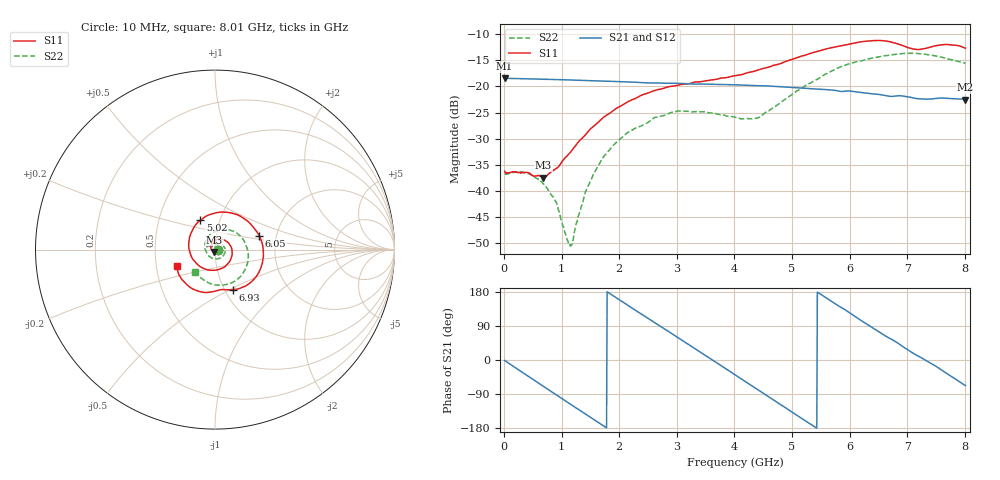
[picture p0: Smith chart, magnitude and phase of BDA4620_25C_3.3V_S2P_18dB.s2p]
!Agilent Technologies,E5071B,MY42404982,A.09.10
!Date: Wed May 06 08:52:32 2026
!Data & Calibration Information:
!Freq	S11:SOLT2(ON)	S21:SOLT2(ON)	S12:SOLT2(ON)	S22:SOLT2(ON)
# Hz S RI R 50
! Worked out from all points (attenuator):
!   801 points, 10 MHz to 8.01 GHz, reference 50 ohm
!   highest |S21| = -18.41 dB at 10 MHz (marker M1); lowest = -22.5 dB at 8.01 GHz (marker M2)
!   lowest |S11| = -37.5 dB at 680 MHz (marker M3), VSWR 1.03, Z = 49.7 - j1.3 ohm
!   |S11| at or under -10 dB: start of sweep to end of sweep
!   |S22| runs from -50.6 to -13.6 dB; largest |S21 - S12| = 0.00059
!   S11 on the Smith chart (normalised r, x): 10 MHz: 1.03, -0.00; 5.02 GHz: 0.81, +0.27; 6.05 GHz: 1.62, +0.27; 6.93 GHz: 1.09, -0.52; 8.01 GHz: 0.64, -0.13
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1e7  0.0154 -0.00104  0.1201 -0.00251  0.1202 -0.00259  0.0144 -0.00056
4.2e8  0.00861 -0.0122  0.0866 -0.0804  0.0867 -0.0806  0.0136 -0.00548
6.8e8  -0.00279 -0.0131  0.0418 -0.1096  0.0419 -0.1097  0.00894 -0.00752
8.9e8  -0.0137 -0.0086  -0.000386 -0.1163  -0.000431 -0.1166  0.00341 -0.00727
1.14e9  -0.0222 0.0058  -0.0492 -0.1043  -0.0494 -0.1044  -0.00257 -0.00184
1.19e9  -0.023 0.0098  -0.058 -0.0993  -0.0582 -0.0995  -0.00329 -8.74e-05
1.35e9  -0.0227 0.0223  -0.0827 -0.0789  -0.0827 -0.079  -0.00497 0.0053
1.58e9  -0.0135 0.0404  -0.1058 -0.0402  -0.1059 -0.0403  -0.0041 0.0148
1.87e9  0.0119 0.0559  -0.1107 0.0155  -0.1109 0.0156  0.00411 0.0259
2.16e9  0.0458 0.0553  -0.0885 0.0662  -0.0885 0.0661  0.0189 0.0312
2.68e9  0.0935 0.00364  -0.00434 0.1077  -0.0043 0.1079  0.0474 0.0193
3.08e9  0.0838 -0.0625  0.0642 0.0852  0.0646 0.0851  0.0575 -0.00966
4.01e9  -0.0881 -0.0909  0.0805 -0.0651  0.0806 -0.0653  -0.0137 -0.049
4.42e9  -0.1443 0.000156  0.0183 -0.0999  0.0182 -0.1  -0.0488 -0.0125
5.02e9  -0.0819 0.1635  -0.0743 -0.0635  -0.0745 -0.0637  -0.0314 0.0795
5.35e9  0.0236 0.2084  -0.094 -0.013  -0.0942 -0.0131  0.0241 0.1072
6.05e9  0.2459 0.0781  -0.0436 0.0783  -0.0437 0.0784  0.1595 0.0528
6.37e9  0.2662 -0.0623  0.00334 0.0851  0.00339 0.0852  0.1846 -0.0186
6.68e9  0.1936 -0.1873  0.0421 0.0686  0.0423 0.0688  0.1742 -0.0964
6.93e9  0.0993 -0.2239  0.0664 0.0459  0.0666 0.0461  0.1398 -0.1521
7.57e9  -0.0887 -0.2327  0.0708 -0.0313  0.0709 -0.0311  -0.0226 -0.1899
8.01e9  -0.2132 -0.0925  0.0284 -0.069  0.0285 -0.0691  -0.109 -0.125
